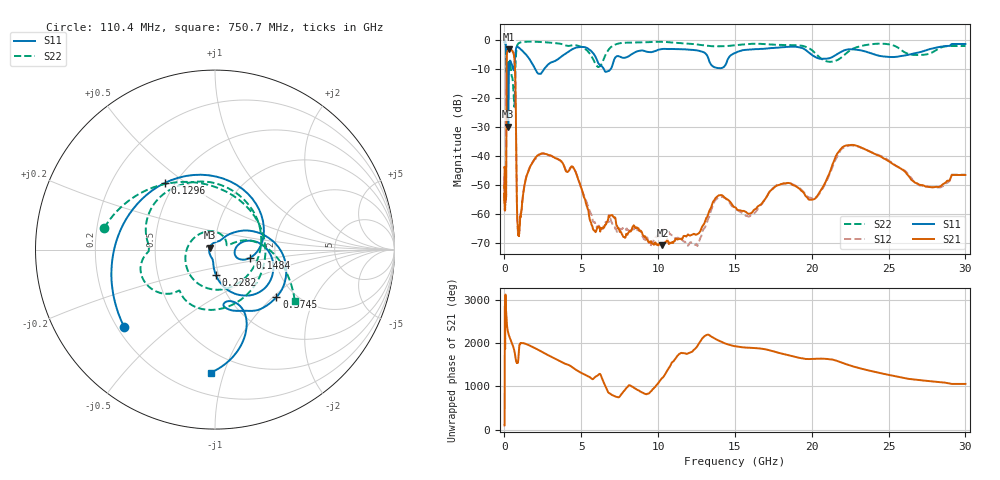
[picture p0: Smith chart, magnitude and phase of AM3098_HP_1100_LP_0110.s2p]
! Date/Time: Thu, Feb 28, 2019 8:44 AM
! Network Analyzer: Agilent Technologies E8364B Rev: A.07.50.67
! Sweep from 0.010 to 30.000 GHz, 1601 Points, Sweep Type: LOG
! Power Supply: 5.023 V, 0.002 A
# Hz S DB R 50
!freq MagS11 AngS11 MagS21 AngS21 MagS12 AngS12 MagS22 AngS22
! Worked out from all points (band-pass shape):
!   1601 points, 10 MHz to 30 GHz, reference 50 ohm
!   highest |S21| = -3.41 dB at 265.1 MHz (marker M1); lowest = -70.7 dB at 10.28 GHz (marker M2)
!   |S21| within 3 dB of the highest: 148.5 MHz to 644.7 MHz (496.2 MHz wide, 125 % of centre)
!   lowest |S11| = -29.9 dB at 246 MHz (marker M3), VSWR 1.07, Z = 47.1 + j0.998 ohm
!   |S11| at or under -10 dB: 205.4 MHz to 298.3 MHz (92.94 MHz wide, 36.9 % of centre); 1.992 GHz to 2.601 GHz (609.2 MHz wide, 26.5 % of centre); 6.451 GHz to 6.933 GHz (481.8 MHz wide, 7.2 % of centre)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
!   |S22| runs from -23.1 to -0.6 dB; largest |S21 - S12| = 0.0089
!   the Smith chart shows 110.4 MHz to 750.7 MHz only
!   S11 on the Smith chart (normalised r, x): 110.4 MHz: 0.23, -0.35; 129.6 MHz: 0.44, +0.42; 148.4 MHz: 1.47, -0.14; 228.2 MHz: 0.97, -0.28; 374.5 MHz: 1.61, -1.05; 750.7 MHz: 0.35, -0.90
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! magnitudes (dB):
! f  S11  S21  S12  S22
! 10 MHz  -0.4  -43.9  -47.1  -0.6
! 38.04 MHz  -0.4  -57.6  -56.1  -0.8
! 110.4 MHz  -3.5  -52.4  -51.6  -4.0
! 129.6 MHz  -6.6  -21.3  -21.4  -10.8
! 144.7 MHz  -11.8  -7.6  -7.5  -9.5
! 148.4 MHz  -14.1  -6.5  -6.4  -9.9
! 228.2 MHz  -16.9  -3.5  -3.5  -8.4
! 246 MHz  -29.9  -3.5  -3.4  -8.7
! 265.1 MHz  -17.1  -3.4  -3.4  -8.5
! 374.5 MHz  -7.3  -3.7  -3.6  -8.3
! 550.5 MHz  -9.9  -4.3  -4.2  -14.8
! 679.2 MHz  -7.2  -9.2  -9.1  -17.5
! 750.7 MHz  -3.3  -29.3  -29.4  -5.5
! 821.5 MHz  -2.4  -59.0  -59.5  -2.2
! 903.4 MHz  -2.7  -65.9  -66.9  -1.4
! 2.084 GHz  -10.9  -40.2  -40.6  -0.8
! 4.48 GHz  -3.2  -44.0  -44.1  -1.9
! 7.926 GHz  -6.1  -66.7  -65.4  -1.1
! 10.28 GHz  -3.3  -70.7  -66.2  -0.8
! 20.1 GHz  -5.6  -54.9  -54.8  -4.1
! 22.56 GHz  -3.4  -36.2  -36.3  -3.5
! 30 GHz  -1.5  -46.5  -46.4  -2.2
